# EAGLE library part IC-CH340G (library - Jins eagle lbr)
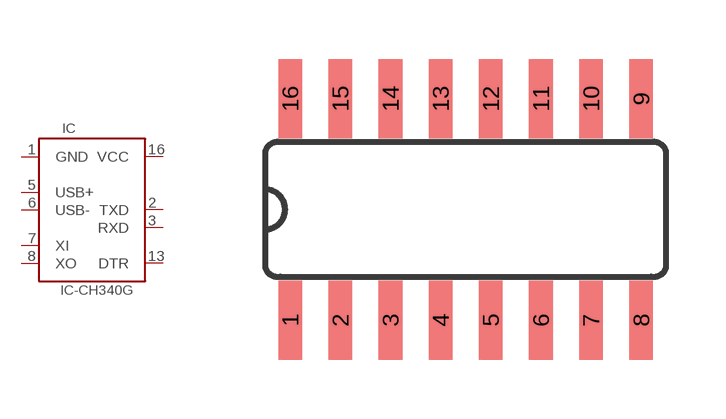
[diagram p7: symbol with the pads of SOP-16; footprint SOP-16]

Designator prefix IC

## IC-CH340G-USB-TTL  [SOP-16]
1  GND
2  TXD
3  RXD
5  USB+
6  USB-
7  XI
8  XO
13  DTR
16  VCC

## Footprint SOP-16 (pad centres in mm)
smd 0.6 x 2: 1 -3.945,-2.76; 2 -2.675,-2.76; 3 -1.405,-2.76; 4 -0.135,-2.76; 5 1.135,-2.76; 6 2.405,-2.76; 7 3.675,-2.76; 8 4.945,-2.76; 9 4.945,2.84; 10 3.675,2.84; 11 2.405,2.84; 12 1.135,2.84; 13 -0.135,2.84; 14 -1.405,2.84; 15 -2.675,2.84; 16 -3.945,2.84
